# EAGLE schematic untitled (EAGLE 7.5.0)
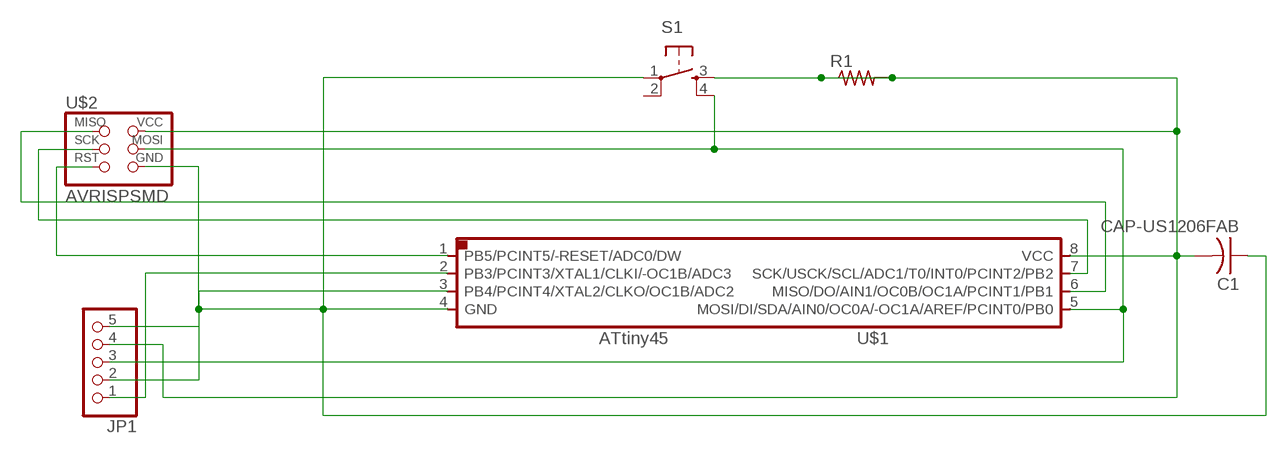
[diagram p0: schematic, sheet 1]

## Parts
C1  CAP-US1206FAB  [C1206FAB]
JP1  PINHD-1X5  [1X05]
R1  RES-US1206FAB  [R1206FAB]
S1  6MM_SWITCH6MM_SWITCH  [6MM_SWITCH]
U$1  ATTINY45SI  [SOIC8]
U$2  AVRISPSMD  [2X03SMD]

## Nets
N$1: C1.1 JP1.5 S1.1(P) U$1.4(GND) U$2.6(GND)
N$2: C1.2 JP1.4 R1.1 R1.2 S1.3(S) U$1.8(VCC) U$2.2(VCC)
N$3: U$1.6(MISO/DO/AIN1/OC0B/OC1A/PCINT1/PB1) U$2.1(MISO)
N$4: U$1.7(SCK/USCK/SCL/ADC1/T0/INT0/PCINT2/PB2) U$2.3(SCK)
N$5: JP1.3 S1.4(S1) U$1.5(MOSI/DI/SDA/AIN0/OC0A/-OC1A/AREF/PCINT0/PB0) U$2.4(MOSI)
N$6: U$1.1(PB5/PCINT5/-RESET/ADC0/DW) U$2.5(RST)
N$7: JP1.2 U$1.3(PB4/PCINT4/XTAL2/CLKO/OC1B/ADC2)
N$8: JP1.1 U$1.2(PB3/PCINT3/XTAL1/CLKI/-OC1B/ADC3)
Unconnected: S1.2(P1)

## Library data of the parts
C1 = fab:CAP-US
JP1 = pinhead:PINHD-1X5: PIN HEADER
R1 = fab:RES-US: Resistor (US Symbol)
S1 = fab:6MM_SWITCH: OMRON SWITCH
U$1 = fab:ATTINY45
U$2 = fab:AVRISP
